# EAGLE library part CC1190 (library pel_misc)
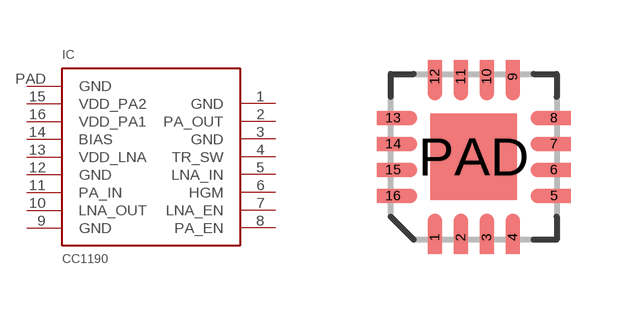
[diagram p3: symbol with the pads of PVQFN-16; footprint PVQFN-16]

Designator prefix IC

## CC1190  [PVQFN-16]
1  GND
2  PA_OUT
3  GND
4  TR_SW
5  LNA_IN
6  HGM
7  LNA_EN
8  PA_EN
9  GND
10  LNA_OUT
11  PA_IN
12  GND
13  VDD_LNA
14  BIAS
15  VDD_PA2
16  VDD_PA1
PAD  GND

## Footprint PVQFN-16 (pad centres in mm)
smd 0.35 x 0.825: 1 -0.975,-2.013; 2 -0.325,-2.013; 3 0.325,-2.013; 4 0.975,-2.013; 9 0.975,2.013; 10 0.325,2.013; 11 -0.325,2.013; 12 -0.975,2.013
smd 0.825 x 0.35: 5 2.013,-0.975; 6 2.013,-0.325; 7 2.013,0.325; 8 2.013,0.975; 13 -2.013,0.975; 14 -2.013,0.325; 15 -2.013,-0.325; 16 -2.013,-0.975
smd 2.16 x 2.16: PAD 0,0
